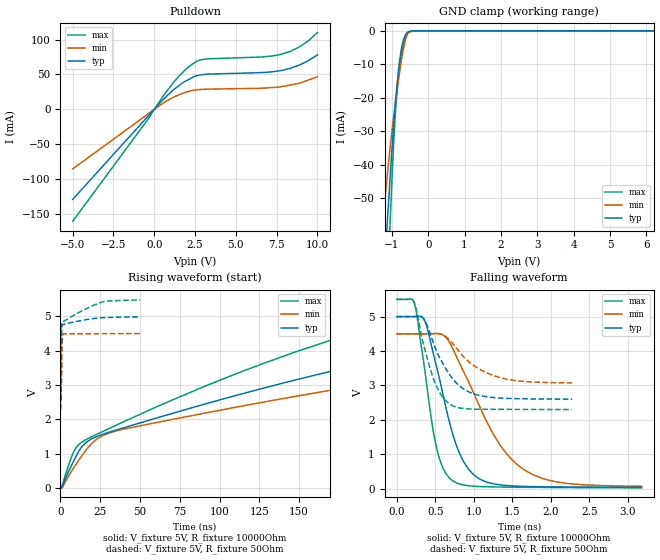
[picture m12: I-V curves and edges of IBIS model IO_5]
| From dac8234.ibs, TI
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|   io_5 Model
[Model]   IO_5
Model_type   I/O_open_drain
Polarity   Non-Inverting
Enable   Active-Low
Vinl = 0.6
Vinh = 2.5
Vmeas = 2.5
Vref = 5
Cref = 15pF
Rref = 10000
|   typ   min   max
|   (nom PVT)   (Fast PVT)   (slow PVT)
|Average
C_comp   4.843e-12   3.910e-12   5.780e-12
|ON state : BUFFER OUTPUT TURNED HIGH
|C_comp   4.951e-12   4.037e-12   5.902e-12
|OFF state: BUFFER in HIGH IMPEDANCE for IOs and 3-state,
|This is BUFFER in LOW state for OUTPUT only type
|C_comp   4.735e-12   3.783e-12   5.659e-12
| Where nom  PVT is Nominal Process, 5V, 42C
|   Fast PVT is Strong Process,  5.5V, -40C
|   Slow PVT is Weak Process,   4.5V, 122C
[Voltage Range]   5   4.5   5.5
|Ambient Temperature   25   105   -40
|Junction Temperature
[Temperature Range]   42   122   -40
[Pullup Reference]   5   4.5   5.5
[Pulldown Reference]   0   0   0
[Power Clamp Reference]   5   4.5   5.5
[GND Clamp Reference]   0   0   0
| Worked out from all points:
|   slope of the pulldown table from 0 to 0.75 V, typ, clamps not added: 40.3 ohm
|   GND clamp passes 1 mA (typ) near -0.61 V on its own axis
|   falling waveform, V_fixture 5V, R_fixture 10000Ohm: 20-80 % time 348ps typ, 626ps min, 224ps max; typ from 5 V to 0.039 V
|   rising waveform, V_fixture 5V, R_fixture 10000Ohm: 20-80 % time 218ns typ, 259ns min, 168ns max; typ from 0.018 V to 4.99 V
|   falling waveform, V_fixture 5V, R_fixture 50Ohm: 20-80 % time 338ps typ, 449ps min, 238ps max; typ from 5 V to 2.6 V
|   rising waveform, V_fixture 5V, R_fixture 50Ohm: 20-80 % time 246ps typ, 305ps min, 1.32ns max; typ from 2.59 V to 4.98 V
[Pulldown]
|   Voltage   I(typ)   I(min)   I(max)
-5V       -128.9mA   -85.22mA   -160.2mA
-413mV    -10.52mA   -7.085mA   -14.99mA
475mV     12.39mA    7.804mA    16.86mA
1.171V    27.87mA    17.2mA     38.46mA
2.227V    44.3mA     26.66mA    63.08mA
2.612V    48.2mA     28.04mA    69.04mA
3.261V    50.49mA    29mA       72.4mA
6.588V    52.68mA    30.36mA    75.04mA
7.766V    55.59mA    32.47mA    78.76mA
8.926V    63.83mA    37.77mA    89.81mA
9.465V    70.11mA    42.18mA    98.62mA
10V       78.11mA    46.56mA    110mA
[GND Clamp]
|   Voltage   I(typ)   I(min)   I(max)
-5V       -915.8mA   -639.1mA   -1.312A
-1.254V   -81.7mA    -58.09mA   -117.5mA
-1.123V   -57.01mA   -43.1mA    -78.65mA
-1.062V   -46.48mA   -36.61mA   -61.35mA
-1.04V    -42.7mA    -34.25mA   -55.6mA
-946.5mV  -27.93mA   -25.45mA   -32.97mA
-853mV    -15.61mA   -17.64mA   -17.74mA
-798mV    -10.12mA   -13.34mA   -11.93mA
-725mV    -4.786mA   -8.086mA   -6.538mA
-633mV    -1.418mA   -2.978mA   -2.099mA
-540mV    -246.6uA   -560.8uA   -419.3uA
10V       0A         0A         0A
[POWER Clamp]
|   Voltage   I(typ)   I(min)   I(max)
-5V       0A         0A         0A
10V       0A         0A         0A
[Ramp]
R_load = 10000
|   typ   min   max
dV/dt_r   2.98906/2.18221e-07   2.68358/2.62485e-07   3.29123/1.67731e-07
dV/dt_f   2.98914/3.50934e-10   2.68489/6.38064e-10   3.29123/2.24468e-10
[Falling Waveform]
V_fixture = 5V
V_fixture_min = 4.5V
V_fixture_max = 5.5V
R_fixture = 10000Ohm
|   Time   V(typ)   V(min)   V(max)
0s        5V         4.5V       5.5V
225ps     5.001V     4.5V       5.419V
350ps     4.933V     4.5V       3.667V
500ps     3.689V     4.508V     1.353V
700ps     1.791V     4.19V      272.8mV
1ns       402.5mV    2.765V     69.57mV
1.325ns   114.1mV    1.319V     47.12mV
1.6ns     68.84mV    633.8mV    40.46mV
2.175ns   48.53mV    161.2mV    31.1mV
3.175ns   38.73mV    67.8mV     22.34mV
[Rising Waveform]
V_fixture = 5V
V_fixture_min = 4.5V
V_fixture_max = 5.5V
R_fixture = 10000Ohm
|   Time   V(typ)   V(min)   V(max)
0s        18.1mV     25.17mV    14.62mV
10.03ns   938mV      705.9mV    1.185V
16.6ns    1.342V     1.132V     1.42V
32.12ns   1.644V     1.622V     1.763V
145.7ns   3.121V     2.65V      3.927V
237.1ns   4.078V     3.346V     5.12V
305.8ns   4.612V     3.788V     5.407V
364.2ns   4.85V      4.092V     5.465V
469.6ns   4.959V     4.387V     5.494V
632.4ns   4.993V     4.471V     5.5V
[Falling Waveform]
V_fixture = 5V
V_fixture_min = 4.5V
V_fixture_max = 5.5V
R_fixture = 50Ohm
|   Time   V(typ)   V(min)   V(max)
0s        5V         4.5V       5.5V
225ps     5.001V     4.5V       5.426V
350ps     4.939V     4.5V       4.165V
475ps     4.233V     4.504V     3.206V
575ps     3.73V      4.492V     2.725V
700ps     3.264V     4.283V     2.442V
925ps     2.822V     3.704V     2.317V
1.275ns   2.643V     3.271V     2.304V
1.6ns     2.612V     3.126V     2.303V
2.275ns   2.601V     3.073V     2.297V
[Rising Waveform]
V_fixture = 5V
V_fixture_min = 4.5V
V_fixture_max = 5.5V
R_fixture = 50Ohm
|   Time   V(typ)   V(min)   V(max)
0s        2.587V     3.06V      2.289V
275ps     2.582V     3.06V      2.343V
325ps     2.581V     3.059V     2.642V
425ps     2.703V     3.056V     3.892V
525ps     3.278V     3.05V      4.598V
750ps     4.524V     3.244V     4.814V
1.125ns   4.747V     4.257V     4.824V
1.725ns   4.761V     4.487V     4.843V
26.15ns   4.958V     4.493V     5.412V
49.98ns   4.983V     4.497V     5.479V
